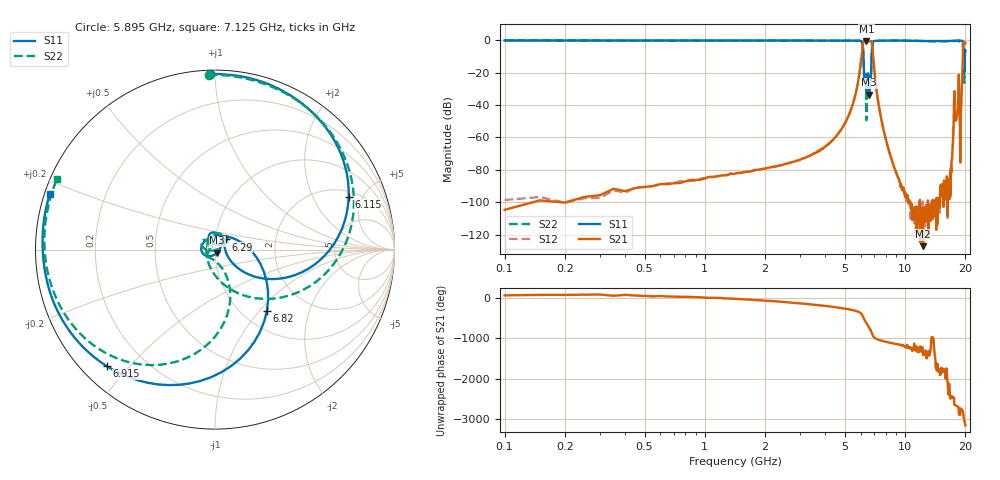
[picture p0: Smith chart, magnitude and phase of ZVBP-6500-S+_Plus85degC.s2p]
! Mini-Circuits
! S2P DATA File Format
! Type: BAND PASS FILTER
! Model: ZVBP-6500-S+
! All S Parameters are in dB deg format
! TEST CONDITIONS: INPUT POWER = 0 dBm @ Temperature = +85deg C
# MHZ S DB R 50
!Frequency  S11 dB  S11 DEG  S21 dB  S21 DEG  S12 dB  S12 DEG  S22 dB  S22 DEG
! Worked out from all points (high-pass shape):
!   1299 points, 100 MHz to 20 GHz, reference 50 ohm
!   highest |S21| = -0.33 dB at 6.405 GHz (marker M1); lowest = -127.2 dB at 12.3 GHz (marker M2)
!   |S21| within 3 dB of the highest: 6.143 GHz to 6.85 GHz (707.1 MHz wide, 10.9 % of centre); 19.49 GHz to end of sweep
!   lowest |S11| = -33.5 dB at 6.625 GHz (marker M3), VSWR 1.04, Z = 51.2 - j1.73 ohm
!   |S11| at or under -10 dB: 6.196 GHz to 6.802 GHz (606.5 MHz wide, 9.33 % of centre); 19.52668 GHz to 19.57448 GHz (47.8 MHz wide, 0.244 % of centre); 19.7 GHz to 19.82 GHz (120.3 MHz wide, 0.609 % of centre)
!   |S22| runs from -49.3 to 0.0 dB; largest |S21 - S12| = 0.0023
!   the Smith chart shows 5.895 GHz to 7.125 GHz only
!   S11 on the Smith chart (normalised r, x): 5.895 GHz: 0.02, +0.97; 6.115 GHz: 2.36, +3.88; 6.29 GHz: 1.12, +0.13; 6.82 GHz: 1.29, -1.10; 6.915 GHz: 0.07, -0.43; 7.125 GHz: 0.02, +0.16
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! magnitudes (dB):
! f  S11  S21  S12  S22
! 100 MHz  0.0  -104.7  -98.6  0.0
! 250 MHz  -0.1  -96.8  -97.5  -0.1
! 600 MHz  -0.1  -88.8  -88.9  -0.1
! 1.45 GHz  -0.1  -81.9  -82.1  -0.1
! 3.45 GHz  -0.1  -70.3  -70.4  -0.2
! 4.925 GHz  -0.1  -52.8  -52.8  -0.2
! 5.895 GHz  -0.2  -21.7  -21.7  -0.2
! 6.115 GHz  -1.9  -5.4  -5.4  -2.0
! 6.29 GHz  -21.6  -0.4  -0.4  -21.6
! 6.405 GHz  -31.1  -0.3  -0.3  -43.0
! 6.505 GHz  -20.4  -0.4  -0.4  -21.3
! 6.625 GHz  -33.5  -0.3  -0.3  -30.3
! 6.82 GHz  -7.0  -1.6  -1.6  -7.0
! 6.915 GHz  -1.1  -9.3  -9.3  -1.1
! 7.125 GHz  -0.3  -26.2  -26.2  -0.3
! 8.275 GHz  -0.1  -67.4  -67.4  -0.2
! 12.3 GHz  -0.3  -127.2  -105.6  -0.4
! 16.8 GHz  -0.3  -80.6  -80.7  -0.5
! 17.7 GHz  -0.2  -46.2  -46.2  -0.4
! 18.95 GHz  -0.2  -48.4  -48.5  -0.3
! 19.55 GHz  -13.1  -1.3  -1.3  -14.0
! 20 GHz  -7.3  -1.7  -1.7  -7.4
